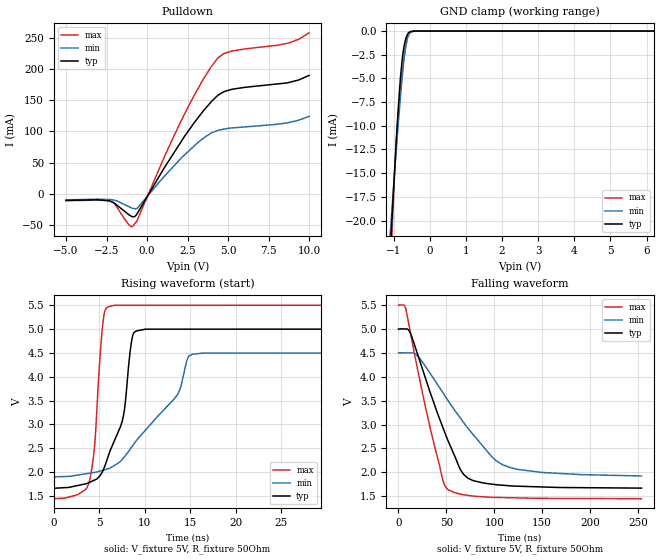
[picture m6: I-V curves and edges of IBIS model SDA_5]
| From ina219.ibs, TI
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|   5V SDA I/O_Open_drain Model
[Model] SDA_5   |Rload = 1k
Model_type I/O_open_drain
| Signals  SDA
Polarity   Non-Inverting
Enable   Active-Low
Vinl = 1.5
Vinh = 3.5
Vmeas = 2.5
Vref = 2.5
Cref = 0pF
Rref = 50
|   typ   min   max
|Average
C_comp   1.6449541E-10   1.4911062E-10   2.4476750E-10
|ON state
|C_comp   2.1193190e-12   2.3639330e-12   1.8543070e-12
|OFF state
|C_comp   3.2687150e-10   2.9585730e-10   4.8768070e-10
[Voltage Range]   5   4.5   5.5
[Temperature Range]   27   85   -25
[Pullup Reference]   5   4.5   5.5
[Pulldown Reference]   -0   -0   -0
[Power Clamp Reference]   5   4.5   5.5
[GND Clamp Reference]   0   0   0
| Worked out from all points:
|   slope of the pulldown table from 0 to 0.75 V, typ, clamps not added: 22.8 ohm
|   GND clamp passes 1 mA (typ) near -0.67 V on its own axis
|   falling waveform, V_fixture 5V, R_fixture 50Ohm: 20-80 % time 36.6ns typ, 56.7ns min, 26.7ns max; typ from 5 V to 1.67 V
|   rising waveform, V_fixture 5V, R_fixture 50Ohm: 20-80 % time 2.3ns typ, 6.03ns min, 880ps max; typ from 1.67 V to 5 V
[Pulldown]
|   Voltage   I(typ)   I(min)   I(max)
-5V       -10.74mA   -10.08mA   -11.25mA
-2.205V   -12.75mA   -9.515mA   -12.54mA
-1.135V   -33.53mA   -20.68mA   -49.43mA
-893mV    -37.08mA   -23.46mA   -52.51mA
-584.9mV  -30.72mA   -22.76mA   -40.99mA
1.052V    41.16mA    27.59mA    58.28mA
2.269V    90.44mA    61.22mA    125.9mA
3.402V    130.6mA    87.5mA     180.8mA
4.333V    157mA      101.2mA    216.9mA
5.235V    167.5mA    105.4mA    228.9mA
8.747V    178.4mA    114.2mA    241.9mA
9.985V    189.7mA    124mA      258mA
[GND Clamp]
|   Voltage   I(typ)   I(min)   I(max)
-5V       -333.3mA   -246mA     -478.3mA
-1.088V   -22.99mA   -21.11mA   -25.81mA
-1.049V   -20.18mA   -19.06mA   -21.96mA
-1.036V   -19.23mA   -18.37mA   -20.72mA
-964.5mV  -14.26mA   -14.58mA   -14.51mA
-903.9mV  -10.24mA   -11.51mA   -10.47mA
-816.8mV  -5.306mA   -7.296mA   -6.481mA
-764.9mV  -3.145mA   -5.033mA   -4.598mA
-676mV    -1.022mA   -1.839mA   -1.97mA
-613.5mV  -347.2uA   -588.3uA   -784.5uA
-547.5mV  -76.59uA   -122.3uA   -198.2uA
9.985V    0A         0A         0A
[POWER Clamp]
|   SCR cell for ESD function. Effects occurr above VDD x 2
|   Voltage   I(typ)   I(min)   I(max)
-5V       0A         0A         0A
0V        0A         0A         0A
10V       0A         0A         0A
[Ramp]
R_load = 50
|   typ   min   max
dV/dt_r   2.0006/2.30868e-009   1.55708/6.0357e-009   2.4316/8.74898e-010
dV/dt_f   1.99852/3.66305e-008   1.54604/5.66826e-008   2.43124/2.66697e-008
[Falling Waveform]
V_fixture = 5V
V_fixture_min = 4.5V
V_fixture_max = 5.5V
R_fixture = 50Ohm
C_fixture = 0F
|   Time   V(typ)   V(min)   V(max)
0s        5V         4.5V       5.5V
7.347ns   5V         4.499V     5.439V
13.65ns   4.846V     4.498V     4.799V
33.21ns   3.665V     4.066V     2.917V
46.42ns   2.933V     3.664V     1.828V
51.5ns    2.672V     3.51V      1.642V
72.6ns    1.876V     2.918V     1.517V
96.92ns   1.754V     2.336V     1.477V
115.7ns   1.719V     2.104V     1.468V
253.7ns   1.669V     1.923V     1.448V
[Rising Waveform]
V_fixture = 5V
V_fixture_min = 4.5V
V_fixture_max = 5.5V
R_fixture = 50Ohm
C_fixture = 0F
|   Time   V(typ)   V(min)   V(max)
0s        1.666V     1.905V     1.447V
3.828ns   1.781V     1.978V     1.759V
4.499ns   1.839V     1.998V     2.595V
5.49ns    2.076V     2.047V     5.268V
6.724ns   2.69V      2.152V     5.492V
7.641ns   3.176V     2.298V     5.492V
8.675ns   4.868V     2.56V      5.492V
10.04ns   4.993V     2.876V     5.492V
16.33ns   4.993V     4.492V     5.493V
253.7ns   5V         4.5V       5.5V
